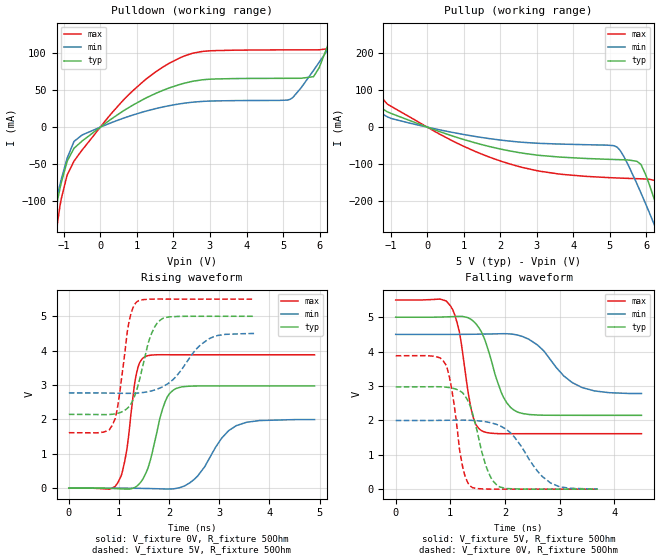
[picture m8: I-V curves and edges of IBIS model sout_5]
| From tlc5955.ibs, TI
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|   sout_5 Model
[Model]   sout_5
Model_type   Output
Polarity   Non-Inverting
Vmeas = 2.5
Vref = 0
Cref = 15pF
Rref = 100
|   typ   min   max
|   (nom PVT)   (fast PVT)   (slow PVT)
C_comp   1.316e-12   1.219e-12   1.501e-12
| Where nom  PVT is Nominal Process, 5V, 27C
|   Fast PVT is Strong Process,  5.5V, -40C
|   Slow PVT is Weak Process,   4.5V, 125C
[Voltage Range]   5   4.5   5.5
|Junction Temperature
[Temperature Range]   27   125   -40
[Pullup Reference]   5   4.5   5.5
[Pulldown Reference]   0   0   0
[Power Clamp Reference]   5   4.5   5.5
[GND Clamp Reference]   0   0   0
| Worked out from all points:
|   slope of the pulldown table from 0 to 0.75 V, typ, clamps not added: 29.4 ohm
|   slope of the pullup table from 0 to 0.75 V, typ, clamps not added: 29.2 ohm
|   falling waveform, V_fixture 5V, R_fixture 50Ohm: 20-80 % time 350ps typ, 592ps min, 231ps max; typ from 5 V to 2.15 V
|   rising waveform, V_fixture 0V, R_fixture 50Ohm: 20-80 % time 307ps typ, 545ps min, 206ps max; typ from 0 V to 2.97 V
|   rising waveform, V_fixture 5V, R_fixture 50Ohm: 20-80 % time 309ps typ, 572ps min, 211ps max; typ from 2.15 V to 5 V
|   falling waveform, V_fixture 0V, R_fixture 50Ohm: 20-80 % time 300ps typ, 537ps min, 208ps max; typ from 2.97 V to 0 V
[Pulldown]
|   Voltage   I(typ)   I(min)   I(max)
-5V       -1.337A    -1.051A    -1.768A
-1.409V   -166.9mA   -142.3mA   -235.8mA
-1.301V   -134.7mA   -118.4mA   -184.8mA
-1.067V   -74.37mA   -69.71mA   -96.08mA
-720.5mV  -28.37mA   -19.15mA   -45.6mA
879.5mV   29.38mA    16.16mA    48.64mA
2.281V    58.93mA    32.15mA    95.51mA
5.202V    65.78mA    37.63mA    104.1mA
5.835V    67.96mA    76.43mA    104.1mA
6.335V    124.5mA    112.4mA    106.2mA
6.676V    171.2mA    137.1mA    160.2mA
10V       567.1mA    361.5mA    890mA
[Pullup]
|   Voltage   I(typ)   I(min)   I(max)
-5V       500.3mA    294.3mA    839.4mA
-4.478V   449.9mA    260.9mA    781mA
-3.095V   294mA      167.1mA    561.9mA
-2.325V   194.7mA    112.3mA    385.5mA
-981.5mV  36.61mA    23.11mA    55.53mA
2.168V    -62.32mA   -36.64mA   -96.36mA
5.192V    -87.33mA   -53.41mA   -136.8mA
5.85V     -100.5mA   -177.2mA   -139.1mA
6.28V     -214mA     -278.1mA   -146mA
6.517V    -288.1mA   -335.8mA   -188.7mA
6.809V    -382.9mA   -408.3mA   -322.4mA
10V       -1.432A    -1.233A    -1.739A
[Ramp]
R_load = 50
|   typ   min   max
dV/dt_r   1.78383/3.05586e-10   1.19695/5.34867e-10   2.32783/2.05655e-10
dV/dt_f   1.71183/3.49457e-10   1.03675/5.90293e-10   2.33258/2.29255e-10
[Falling Waveform]
V_fixture = 5V
V_fixture_min = 4.5V
V_fixture_max = 5.5V
R_fixture = 50Ohm
|   Time   V(typ)   V(min)   V(max)
0s        5V         4.5V       5.5V
1.006ns   5.014V     4.499V     5.321V
1.166ns   5.023V     4.5V       4.575V
1.399ns   4.913V     4.504V     2.206V
1.573ns   4.562V     4.508V     1.698V
1.952ns   2.744V     4.52V      1.612V
2.212ns   2.257V     4.487V     1.612V
2.593ns   2.155V     4.195V     1.612V
3.413ns   2.147V     2.954V     1.612V
4.499ns   2.147V     2.781V     1.612V
[Rising Waveform]
V_fixture = 0V
V_fixture_min = 0V
V_fixture_max = 0V
R_fixture = 50Ohm
|   Time   V(typ)   V(min)   V(max)
0s        1.601nV    8.788nV    1.176nV
981ps     -15.18mV   885.9uV    168mV
1.148ns   -26.15mV   -261.6uV   1.052V
1.346ns   46.96mV    -3.892mV   3.32V
1.496ns   318.4mV    -7.63mV    3.804V
1.919ns   2.512V     -23.27mV   3.881V
2.137ns   2.899V     -8.078mV   3.88V
2.569ns   2.972V     356.1mV    3.88V
3.337ns   2.973V     1.818V     3.88V
4.899ns   2.973V     1.995V     3.88V
[Rising Waveform]
V_fixture = 5V
V_fixture_min = 4.5V
V_fixture_max = 5.5V
R_fixture = 50Ohm
|   Time   V(typ)   V(min)   V(max)
0s        2.147V     2.771V     1.613V
685ps     2.139V     2.769V     1.629V
868ps     2.15V      2.765V     1.835V
978ps     2.179V     2.762V     2.414V
1.198ns   2.367V     2.758V     4.819V
1.355ns   2.863V     2.765V     5.419V
1.641ns   4.471V     2.827V     5.499V
1.873ns   4.937V     2.952V     5.5V
2.789ns   5V         4.34V      5.5V
3.699ns   5V         4.5V       5.5V
[Falling Waveform]
V_fixture = 0V
V_fixture_min = 0V
V_fixture_max = 0V
R_fixture = 50Ohm
|   Time   V(typ)   V(min)   V(max)
0s        2.973V     1.996V     3.879V
720ps     2.979V     1.999V     3.861V
925ps     2.965V     2.002V     3.601V
1.037ns   2.937V     2.005V     2.797V
1.233ns   2.785V     2.007V     595.4mV
1.395ns   2.265V     2V         57.03mV
1.658ns   654.3mV    1.957V     4.127mV
1.88ns    85.46mV    1.863V     -87.59uV
2.837ns   101uV      177.1mV    67.2uV
3.699ns   107.5uV    8.39mV     39.67uV
